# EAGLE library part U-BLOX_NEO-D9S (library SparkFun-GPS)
u-blox NEO-D9S The NEO-D9S can receive the data stream of a GNSS correction service, broadcast via satellite L band and compliant to the specification the product is designed for. Integrated with a high precision GNSS receiver, such as from the u-blox F9 platform, it enables the positioning system to reach down to centimeter-level accuracy.
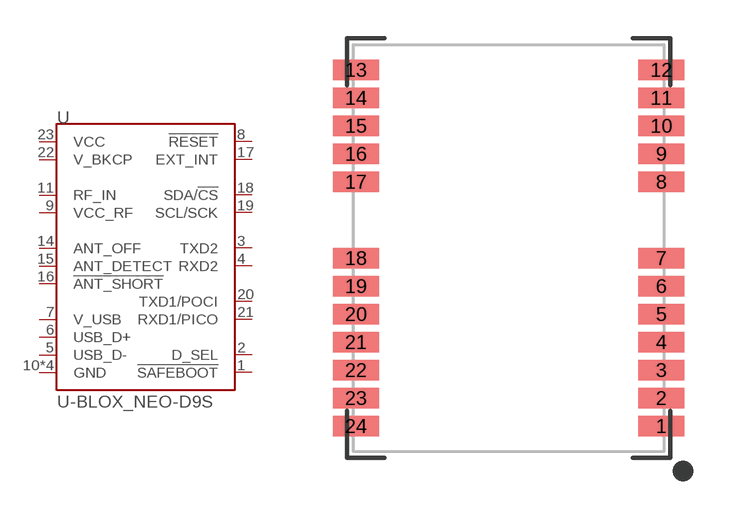
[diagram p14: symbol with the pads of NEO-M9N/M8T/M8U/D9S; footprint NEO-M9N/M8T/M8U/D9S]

Designator prefix U

## U-BLOX_NEO-D9S-00B (PROD_ID: IC-16579)  [NEO-M9N/M8T/M8U/D9S]
1  !SAFEBOOT!  in
2  D_SEL  in
3  TXD2  out
4  RXD2  in
5  USB_D-
6  USB_D+
7  V_USB  pwr
8  !RESET!  in
9  VCC_RF  out
10  GND  pwr
11  RF_IN  in
12  GND  pwr
13  GND  pwr
14  ANT_OFF  out
15  ANT_DETECT  in
16  !ANT_SHORT!  out
17  EXT_INT  in
18  SDA/!CS!
19  SCL/SCK
20  TXD1/POCI  out
21  RXD1/PICO  in
22  V_BKCP  pwr
23  VCC  pwr
24  GND  pwr

## Footprint NEO-M9N/M8T/M8U/D9S (pad centres in mm)
u-blox NEO-M9N/M8T/M8U/D9S Module Mechanical Specifications Overall: 12.2mm x 16.0mm Pad Pitch: 1.1mm Pad Width: .8mm Pad Length: .9mm Number of Pins: 24
smd 1.8 x 0.8: 1 6,-7; 2 6,-5.9; 3 6,-4.8; 4 6,-3.7; 5 6,-2.6; 6 6,-1.5; 7 6,-0.4; 8 6,2.6; 9 6,3.7; 10 6,4.8; 11 6,5.9; 12 6,7; 13 -6,7; 14 -6,5.9; 15 -6,4.8; 16 -6,3.7; 17 -6,2.6; 18 -6,-0.4; 19 -6,-1.5; 20 -6,-2.6; 21 -6,-3.7; 22 -6,-4.8; 23 -6,-5.9; 24 -6,-7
